| IBIS file stm32n657_vfbga198.ibs
[IBIS ver] 4.2
[File name] stm32n657_vfbga198.ibs
[File Rev] 1.1
[Date] 20-09-2024
[Source] Data Created at STMicroelectronics
[Notes]  File originated from ELDO simulations.
[Disclaimer]  This information is for modeling purpose only and is
   not guaranteed. The information is subject to change without
   notice.
[Copyright] Copyright 2024 STMicroelectronics Inc.
|   Component stm32n657_vfbga198
[Component] stm32n657_vfbga198
[Manufacturer] STMicroelectronics
[Package]
| variable   typ   min   max
R_pkg  0  NA  NA
L_pkg  0  NA  NA
C_pkg  0  NA  NA
[Pin]   signal_name   model_name
A1  PDR_ON  nc
A2  OTG2_HSDP  USB2_HS_IBIS
A3  NC  nc
A4  OTG1_HSDP  USB2_HS_IBIS
A5  PH0-OSC_IN  isudq_tt
A6  PC10  io8_tt_i3c
A7  PC7  io8_tt
A8  PE11  io8_tt
A9  PE15  io8_tt_i3c
A10  PD6  io8_tt
A11  PD12  io8_tt
A12  PD3  io8_tt_i3c
A13  PE10  io8_tt
A14  PB3  io8_tt
A15  VSS  gnd
B1  PC15-OSC32_OUT  io8_tt_sw
B2  OTG2_HSDM  USB2_HS_IBIS
B3  VDD33USB  power
B4  OTG1_HSDM  USB2_HS_IBIS
B5  PH1-OSC_OUT  isudq_tt
B6  PC9  io8_tt_i3c
B7  PC6  io8_tt
B8  PE14  io8_tt_i3c
B9  PE13  io8_tt_i3c
B10  PD7  io8_tt
B11  PD1  io8_tt
B12  PD4  io8_tt_i3c
B13  PD8  io8_tt
B14  PD11  io8_tt_i3c
B15  PE2  io8_tt
C1  PC14-OSC32_IN  io8_tt_sw
C2  NC  nc
C3  VDDA18USB  power
C4  OTG1_ID  nc
C5  OTG1_TXRTUNE  nc
C6  PC8  io8_tt_i3c
C7  PC1  io8_tt_i3c
C8  PE5  io8_tt_i3c
C9  PE12  io8_tt
C10  PD10  io8_tt
C11  PD0  io8_tt
C12  PE8  io8_tt
C13  PD5  io8_tt
C14  PE0  io8_tt
C15  PE3  io8_tt
D1  VBAT  power
D2  OTG2_ID  nc
D3  OTG2_TXRTUNE  nc
D4  UCPD1_CC1  nc
D5  UCPD1_CC2  nc
D6  PC11  io8_tt_i3c
D7  PH9  io8_tt_i3c
D8  PE6  io8_tt_i3c
D9  PD2  io8_tt
D10  PE7  io8_tt
D11  PD15  io8_tt_i3c
D12  PE9  io8_tt
D13  PE1  io8_tt
D14  PB6  io8_tt
D15  PB0  io8_tt
E1  V08CAP  nc
E2  VFBSMPS  nc
E3  BOOT0  isudq_tt
E4  NRST  ioreset_tt_v18_1v8
E5  VDDA18AON  nc
E6  PC12  io8_tt
E7  PH2  io8_tt
E8  VSS  gnd
E9  VDDIO4  power
E10  VDDIO4  power
E11  PD14  io8_tt_i3c
E12  PB7  io8_tt
E13  PD9  io8_tt
E14  PP2  io8_tt
E15  PP4  io8_tt
F1  VDDA18PMU  nc
F2  VSSAPMU  nc
F3  PWR_ON  io8_tt
F4  PC13  io8_tt_tamp
F5  VSSAON  nc
F11  PD13  io8_tt
F12  PO1  io8_tt
F13  PP3  io8_tt
F14  PO5  io8_tt
F15  PO4  io8_tt
G1  VSSSMPS  nc
G2  VSSSMPS  nc
G3  VSSSMPS  nc
G4  VSSSMPS  nc
G11  VSS  gnd
G12  PO0  io8_tt
G13  PP6  io8_tt
G14  PP0  io8_tt
G15  PP5  io8_tt
H1  VLXSMPS  nc
H2  VLXSMPS  nc
H3  VLXSMPS  nc
H4  VLXSMPS  nc
H11  VDD  power
H12  VDD  power
H13  PP1  io8_tt
H14  PP7  io8_tt
H15  PO2  io8_tt
J1  VDDSMPS  nc
J2  VDDSMPS  nc
J3  VDDSMPS  nc
J4  VDDSMPS  nc
J5  VDDA18PLL  nc
J11  VDDIO2  power
J12  VDDIO2  power
J13  VDD  power
J14  PN4  io8_tt
J15  PN8  io8_tt
K1  PF4  io8_tt
K2  PF6  io8_tt
K3  PF10  io8_tt
K4  PG6  io8_tt
K5  PG5  io8_tt
K11  VDDIO3  power
K12  PN1  io8_tt
K13  PN5  io8_tt
K14  PN7  io8_tt
K15  PN6  io8_tt
L1  PF5  io8_tt
L2  PF3  io8_tt
L3  PF2  io8_tt
L4  PF14  io8_tt
L5  VSS  gnd
L6  VDDCORE  nc
L7  VDDCORE  nc
L8  VDDCORE  nc
L9  VDDCORE  nc
L10  VSS  gnd
L11  VDDIO3  power
L12  PN12  io8_tt
L13  PN9  io8_tt
L14  PN2  io8_tt
L15  PN10  io8_tt
M1  PF15  io8_tt
M2  PF7  io8_tt
M3  PF8  io8_tt
M4  PF9  io8_tt
M5  VSSA  nc
M6  VDDA18ADC  nc
M7  PG15  io8_tt
M8  PG14  io8_tt
M9  PA9  io8_tt_i3c
M10  PA6  io8_tt_i3c
M11  PA1  io8_tt
M12  PB11  io8_tt_i3c
M13  PN0  io8_tt
M14  PN11  io8_tt
M15  PN3  io8_tt
N1  PF11  io8_tt
N2  PF1  io8_tt
N3  PF12  io8_tt
N4  PF0  io8_tt
N5  CSI_REXT  nc
N6  VDDCSI  nc
N7  PA12  io8_tt
N8  PA11  io8_tt
N9  PA8  io8_tt_i3c
N10  PG13  io8_tt
N11  PA0  io8_tt
N12  PB10  io8_tt_i3c
N13  PB4  io8_tt
N14  PG8  io8_tt
N15  PA3  io8_tt
P1  PF13  io8_tt
P2  PG4  io8_tt
P3  VREFM  nc
P4  CSI_D1N  DPHY_IBIS_L1
P5  CSI_CKN  DPHY_IBIS_L1
P6  CSI_D0N  DPHY_IBIS_L1
P7  VDDA18CSI  power
P8  PA10  io8_tt
P9  PA2  io8_tt
P10  PG12  io8_tt
P11  PG10  io8_tt
P12  PG2  io8_tt
P13  PA7  io8_tt
P14  PG11  io8_tt
P15  PG0  io8_tt
R1  VSS  gnd
R2  PG3  io8_tt
R3  VREFP  nc
R4  CSI_D1P  DPHY_IBIS_L1
R5  CSI_CKP  DPHY_IBIS_L1
R6  CSI_D0P  DPHY_IBIS_L1
R7  PA14  io8_tt
R8  PA13  io8_tt
R9  PA5  io8_tt_i3c
R10  PG1  io8_tt
R11  PB12  io8_tt_i3c
R12  PB5  io8_tt_i3c
R13  PA15  io8_tt
R14  PG9  io8_tt
R15  VSS  gnd
[Package Model]   486-fcvfbga-10x10-198-240308
[Pin Mapping]   pulldown_ref   pullup_ref   | Comment
A1  nc  nc
A2  gnd  VDD33USB
A3  nc  nc
A4  gnd  VDD33USB
A5  gnd  VDD
A6  gnd  VDDIO4
A7  gnd  VDDIO4
A8  gnd  VDD
A9  gnd  VDD
A10  gnd  VDD
A11  gnd  VDD
A12  gnd  VDD
A13  gnd  VDD
A14  gnd  VDD
A15  gnd  nc
B1  gnd  VSW
B2  gnd  VDD33USB
B3  nc  VDD33USB
B4  gnd  VDD33USB
B5  gnd  VDD
B6  gnd  VDDIO4
B7  gnd  VDDIO4
B8  gnd  VDD
B9  gnd  VDD
B10  gnd  VDD
B11  gnd  VDD
B12  gnd  VDD
B13  gnd  VDD
B14  gnd  VDD
B15  gnd  VDD
C1  gnd  VSW
C2  nc  nc
C3  nc  VDDA18USB
C4  nc  nc
C5  nc  nc
C6  gnd  VDDIO4
C7  gnd  VDDIO4
C8  gnd  VDD
C9  gnd  VDD
C10  gnd  VDD
C11  gnd  VDD
C12  gnd  VDD
C13  gnd  VDD
C14  gnd  VDD
C15  gnd  VDD
D1  nc  VSW
D2  nc  nc
D3  nc  nc
D4  nc  nc
D5  nc  nc
D6  gnd  VDDIO4
D7  gnd  VDDIO4
D8  gnd  VDD
D9  gnd  VDD
D10  gnd  VDD
D11  gnd  VDD
D12  gnd  VDD
D13  gnd  VDD
D14  gnd  VDD
D15  gnd  VDD
E1  nc  nc
E2  nc  nc
E3  gnd  VDD
E4  gnd  VDD
E5  nc  nc
E6  gnd  VDDIO4
E7  gnd  VDDIO4
E8  gnd  nc
E9  nc  VDDIO4
E10  nc  VDDIO4
E11  gnd  VDD
E12  gnd  VDD
E13  gnd  VDD
E14  gnd  VDDIO2
E15  gnd  VDDIO2
F1  nc  nc
F2  nc  nc
F3  gnd  VDD
F4  gnd  VSW
F5  nc  nc
F11  gnd  VDD
F12  gnd  VDDIO2
F13  gnd  VDDIO2
F14  gnd  VDDIO2
F15  gnd  VDDIO2
G1  nc  nc
G2  nc  nc
G3  nc  nc
G4  nc  nc
G11  gnd  nc
G12  gnd  VDDIO2
G13  gnd  VDDIO2
G14  gnd  VDDIO2
G15  gnd  VDDIO2
H1  nc  nc
H2  nc  nc
H3  nc  nc
H4  nc  nc
H11  nc  VDD
H12  nc  VDD
H13  gnd  VDDIO2
H14  gnd  VDDIO2
H15  gnd  VDDIO2
J1  nc  nc
J2  nc  nc
J3  nc  nc
J4  nc  nc
J5  nc  nc
J11  nc  VDDIO2
J12  nc  VDDIO2
J13  nc  VDD
J14  gnd  VDDIO3
J15  gnd  VDDIO3
K1  gnd  VDD
K2  gnd  VDD
K3  gnd  VDD
K4  gnd  VDD
K5  gnd  VDD
K11  nc  VDDIO3
K12  gnd  VDDIO3
K13  gnd  VDDIO3
K14  gnd  VDDIO3
K15  gnd  VDDIO3
L1  gnd  VDD
L2  gnd  VDD
L3  gnd  VDD
L4  gnd  VDD
L5  gnd  nc
L6  nc  nc
L7  nc  nc
L8  nc  nc
L9  nc  nc
L10  gnd  nc
L11  nc  VDDIO3
L12  gnd  VDDIO3
L13  gnd  VDDIO3
L14  gnd  VDDIO3
L15  gnd  VDDIO3
M1  gnd  VDD
M2  gnd  VDD
M3  gnd  VDD
M4  gnd  VDD
M5  nc  nc
M6  nc  nc
M7  gnd  VDD
M8  gnd  VDD
M9  gnd  VDD
M10  gnd  VDD
M11  gnd  VDD
M12  gnd  VDD
M13  gnd  VDDIO3
M14  gnd  VDDIO3
M15  gnd  VDDIO3
N1  gnd  VDD
N2  gnd  VDD
N3  gnd  VDD
N4  gnd  VDD
N5  nc  nc
N6  nc  nc
N7  gnd  VDD
N8  gnd  VDD
N9  gnd  VDD
N10  gnd  VDD
N11  gnd  VDD
N12  gnd  VDD
N13  gnd  VDD
N14  gnd  VDD
N15  gnd  VDD
P1  gnd  VDD
P2  gnd  VDD
P3  nc  nc
P4  gnd  VDDA18CSI
P5  gnd  VDDA18CSI
P6  gnd  VDDA18CSI
P7  nc  VDDA18CSI
P8  gnd  VDD
P9  gnd  VDD
P10  gnd  VDD
P11  gnd  VDD
P12  gnd  VDD
P13  gnd  VDD
P14  gnd  VDD
P15  gnd  VDD
R1  gnd  nc
R2  gnd  VDD
R3  nc  nc
R4  gnd  VDDA18CSI
R5  gnd  VDDA18CSI
R6  gnd  VDDA18CSI
R7  gnd  VDD
R8  gnd  VDD
R9  gnd  VDD
R10  gnd  VDD
R11  gnd  VDD
R12  gnd  VDD
R13  gnd  VDD
R14  gnd  VDD
R15  gnd  nc
[Diff Pin]  inv_pin  vdiff  tdelay_typ  tdelay_min  tdelay_max
R5  P5  NA  NA  NA  NA
R6  P6  NA  NA  NA  NA
R4  P4  NA  NA  NA  NA
A4  B4  NA  NA  NA  NA
A2  B2  NA  NA  NA  NA
[Model Selector] DPHY_IBIS_L1
DPHY_RX_2P5G_L1   DPHY HSRX model at 2.5Gbps for lane 1
DPHY_RX_1P5G_L1   DPHY HSRX model at 1.5Gbps for lane 1
[Model Selector] io8_tt
io8_tt_ls_3v3 "GPIO - 3V tolerant - low speed - 3.3V range"
io8_tt_ms_3v3 "GPIO - 3V tolerant - med speed - 3.3V range"
io8_tt_fs_3v3 "GPIO - 3V tolerant - fast speed - 3.3V range"
io8_tt_hs_3v3 "GPIO - 3V tolerant - high speed - 3.3V range"
io8_tt_hslv_ls_1v8 "GPIO low voltage optimization - 3V tolerant - low speed - 1.8V range"
io8_tt_hslv_ms_1v8 "GPIO low voltage optimization - 3V tolerant - med speed - 1.8V range"
io8_tt_hslv_fs_1v8 "GPIO low voltage optimization - 3V tolerant - fast speed - 1.8V range"
io8_tt_hslv_hs_1v8 "GPIO low voltage optimization - 3V tolerant - high speed - 1.8V range"
[Model Selector] io8_tt_i3c
io8_tt_ls_3v3 "GPIO - 3V tolerant - low speed - 3.3V range"
io8_tt_ms_3v3 "GPIO - 3V tolerant - med speed - 3.3V range"
io8_tt_fs_3v3 "GPIO - 3V tolerant - fast speed - 3.3V range"
io8_tt_hs_3v3 "GPIO - 3V tolerant - high speed - 3.3V range"
io8_tt_hslv_ls_1v8 "GPIO low voltage optimization - 3V tolerant - low speed - 1.8V range"
io8_tt_hslv_ms_1v8 "GPIO low voltage optimization - 3V tolerant - med speed - 1.8V range"
io8_tt_hslv_fs_1v8 "GPIO low voltage optimization - 3V tolerant - fast speed - 1.8V range"
io8_tt_hslv_hs_1v8 "GPIO low voltage optimization - 3V tolerant - high speed - 1.8V range"
io8_tt_i3c_ls_3v3 "GPIO with I3C open-drain - 3V tolerant - low speed - 3.3V range"
io8_tt_i3c_ms_3v3 "GPIO with I3C open-drain - 3V tolerant - med speed - 3.3V range"
io8_tt_i3c_fs_3v3 "GPIO with I3C open-drain - 3V tolerant - fast speed - 3.3V range"
io8_tt_i3c_hs_3v3 "GPIO with I3C open-drain - 3V tolerant - high speed - 3.3V range"
io8_tt_hslv_i3c_ls_1v8 "GPIO low voltage optimization with I3C open-drain - 3V tolerant - low speed - 1.8V range"
io8_tt_hslv_i3c_ms_1v8 "GPIO low voltage optimization with I3C open-drain - 3V tolerant - med speed - 1.8V range"
io8_tt_hslv_i3c_fs_1v8 "GPIO low voltage optimization with I3C open-drain - 3V tolerant - fast speed - 1.8V range"
io8_tt_hslv_i3c_hs_1v8 "GPIO low voltage optimization with I3C open-drain - 3V tolerant - high speed - 1.8V range"
io8_tt_i3c_fmp_3v3 "GPIO with I3C fm+ open-drain - 3V tolerant - 3.3V range"
[Model Selector] io8_tt_sw
io8_tt_sw_3v3 "Input Buffer - 3V tolerant - 3.3V range"
io8_tt_sw_1v8 "Input Buffer - 3V tolerant - 1.8V range"
[Model Selector] io8_tt_tamp
io8_tt_ls_3v3 "GPIO - 3V tolerant - low speed - 3.3V range"
io8_tt_ms_3v3 "GPIO - 3V tolerant - med speed - 3.3V range"
io8_tt_fs_3v3 "GPIO - 3V tolerant - fast speed - 3.3V range"
io8_tt_hs_3v3 "GPIO - 3V tolerant - high speed - 3.3V range"
io8_tt_hslv_ls_1v8 "GPIO low voltage optimization - 3V tolerant - low speed - 1.8V range"
io8_tt_hslv_ms_1v8 "GPIO low voltage optimization - 3V tolerant - med speed - 1.8V range"
io8_tt_hslv_fs_1v8 "GPIO low voltage optimization - 3V tolerant - fast speed - 1.8V range"
io8_tt_hslv_hs_1v8 "GPIO low voltage optimization - 3V tolerant - high speed - 1.8V range"
io8_tt_tamp_3v3 "IO tamper - 3V tolerant - 3.3V range"
io8_tt_tamp_1v8 "IO tamper - 3V tolerant - 1.8V range"
|[Model Selector] ioreset_tt_v18
|ioreset_tt_v18_1v8 "Reset PAD - 3V tolerant - 1.8V range"
[Model Selector] isudq_tt
isudq_tt_3v3 "Input Buffer - 3V tolerant - 3.3V range"
isudq_tt_1v8 "Input Buffer - 3V tolerant - 1.8V range"
[Model Selector] USB2_HS_IBIS
USB2_HSRX   USB2 HSRX model
USB2_HSTX_00_0_01_0011_11   TuningBits_AMP_PULSE_RISE_REF_XV=00_0_01_0011_11
USB2_HSTX_00_0_10_0101_11   TuningBits_AMP_PULSE_RISE_REF_XV=00_0_10_0101_11
USB2_HSTX_00_0_11_0111_11   TuningBits_AMP_PULSE_RISE_REF_XV=00_0_11_0111_11
USB2_HSTX_00_1_01_0011_11   TuningBits_AMP_PULSE_RISE_REF_XV=00_1_01_0011_11
USB2_HSTX_00_1_10_0101_11   TuningBits_AMP_PULSE_RISE_REF_XV=00_1_10_0101_11
USB2_HSTX_00_1_11_0111_11   TuningBits_AMP_PULSE_RISE_REF_XV=00_1_11_0111_11
USB2_HSTX_01_0_01_0011_11   TuningBits_AMP_PULSE_RISE_REF_XV=01_0_01_0011_11
USB2_HSTX_01_0_10_0101_11   TuningBits_AMP_PULSE_RISE_REF_XV=01_0_10_0101_11
USB2_HSTX_01_0_11_0111_11   TuningBits_AMP_PULSE_RISE_REF_XV=01_0_11_0111_11
USB2_HSTX_01_1_01_0011_11   TuningBits_AMP_PULSE_RISE_REF_XV=01_1_01_0011_11
USB2_HSTX_01_1_10_0101_11   TuningBits_AMP_PULSE_RISE_REF_XV=01_1_10_0101_11
USB2_HSTX_01_1_11_0111_11   TuningBits_AMP_PULSE_RISE_REF_XV=01_1_11_0111_11
USB2_HSTX_10_0_01_0011_11   TuningBits_AMP_PULSE_RISE_REF_XV=10_0_01_0011_11
USB2_HSTX_10_0_10_0101_11   TuningBits_AMP_PULSE_RISE_REF_XV=10_0_10_0101_11
USB2_HSTX_10_0_11_0111_11   TuningBits_AMP_PULSE_RISE_REF_XV=10_0_11_0111_11
USB2_HSTX_10_1_01_0011_11   TuningBits_AMP_PULSE_RISE_REF_XV=10_1_01_0011_11
USB2_HSTX_10_1_10_0101_11   TuningBits_AMP_PULSE_RISE_REF_XV=10_1_10_0101_11
USB2_HSTX_10_1_11_0111_11   TuningBits_AMP_PULSE_RISE_REF_XV=10_1_11_0111_11
[Define Package Model]  486-fcvfbga-10x10-198-240308
[Manufacturer]  unknown
[OEM]  unknown
[Description]  unknown
[Number Of Pins]  175
[Pin Numbers]
| Pin Name Terminal   Net Name   Starting Node   Ending Node
E3 | BOOT0
P5 | CSI_CKN
R5 | CSI_CKP
P6 | CSI_D0N
R6 | CSI_D0P
P4 | CSI_D1N
R4 | CSI_D1P
N5 | CSI_REXT
E4 | NRST
B4 | OTG1_HSDM
A4 | OTG1_HSDP
C4 | OTG1_ID
C5 | OTG1_TXRTUNE
A3 | NC
B2 | OTG2_HSDM
A2 | OTG2_HSDP
D2 | OTG2_ID
D3 | OTG2_TXRTUNE
C2 | NC
N11 | PA0
M11 | PA1
P9 | PA2
N15 | PA3
R9 | PA5
M10 | PA6
P13 | PA7
N9 | PA8
M9 | PA9
P8 | PA10
N8 | PA11
N7 | PA12
R8 | PA13
R7 | PA14
R13 | PA15
D15 | PB0
A14 | PB3
N13 | PB4
R12 | PB5
D14 | PB6
E12 | PB7
N12 | PB10
M12 | PB11
R11 | PB12
C7 | PC1
B7 | PC6
A7 | PC7
C6 | PC8
B6 | PC9
A6 | PC10
D6 | PC11
E6 | PC12
F4 | PC13
C1 | PC14-OSC32_IN
B1 | PC15-OSC32_OUT
C11 | PD0
B11 | PD1
D9 | PD2
A12 | PD3
B12 | PD4
C13 | PD5
A10 | PD6
B10 | PD7
B13 | PD8
E13 | PD9
C10 | PD10
B14 | PD11
A11 | PD12
F11 | PD13
E11 | PD14
D11 | PD15
A1 | PDR_ON
C14 | PE0
D13 | PE1
B15 | PE2
C15 | PE3
C8 | PE5
D8 | PE6
D10 | PE7
C12 | PE8
D12 | PE9
A13 | PE10
A8 | PE11
C9 | PE12
B9 | PE13
B8 | PE14
A9 | PE15
N4 | PF0
N2 | PF1
L3 | PF2
L2 | PF3
K1 | PF4
L1 | PF5
K2 | PF6
M2 | PF7
M3 | PF8
M4 | PF9
K3 | PF10
N1 | PF11
N3 | PF12
P1 | PF13
L4 | PF14
M1 | PF15
P15 | PG0
R10 | PG1
P12 | PG2
R2 | PG3
P2 | PG4
K5 | PG5
K4 | PG6
N14 | PG8
R14 | PG9
P11 | PG10
P14 | PG11
P10 | PG12
N10 | PG13
M8 | PG14
M7 | PG15
A5 | PH0-OSC_IN
B5 | PH1-OSC_OUT
E7 | PH2
D7 | PH9
M13 | PN0
K12 | PN1
L14 | PN2
M15 | PN3
J14 | PN4
K13 | PN5
K15 | PN6
K14 | PN7
J15 | PN8
L13 | PN9
L15 | PN10
M14 | PN11
L12 | PN12
G12 | PO0
F12 | PO1
H15 | PO2
F15 | PO4
F14 | PO5
G14 | PP0
H13 | PP1
E14 | PP2
F13 | PP3
E15 | PP4
G15 | PP5
G13 | PP6
H14 | PP7
F3 | PWR_ON
D4 | UCPD1_CC1
D5 | UCPD1_CC2
E1 | V08CAP
D1 | VBAT
B3 | VDD33USB
H11 | VDD
M6 | VDDA18ADC
E5 | VDDA18AON
P7 | VDDA18CSI
J5 | VDDA18PLL
F1 | VDDA18PMU
C3 | VDDA18USB
L6 | VDDCORE
N6 | VDDCSI
J11 | VDDIO2
K11 | VDDIO3
E9 | VDDIO4
J1 | VDDSMPS
E2 | VFBSMPS
H1 | VLXSMPS
P3 | VREFM
R3 | VREFP
A15 | VSS
M5 | VSSA
F5 | VSSAON
F2 | VSSAPMU
G1 | VSSSMPS
|[Merged Pins]  H11
|H12  |  VDD
|J13  |  VDD
|[Merged Pins]  L6
|L7  |  VDDCORE
|L8  |  VDDCORE
|L9  |  VDDCORE
|[Merged Pins]  J11
|J12  |  VDDIO2
|[Merged Pins]  K11
|L11  |  VDDIO3
|[Merged Pins]  E9
|E10  |  VDDIO4
|[Merged Pins]  J1
|J2  |  VDDSMPS
|J3  |  VDDSMPS
|J4  |  VDDSMPS
|[Merged Pins]  H1
|H2  |  VLXSMPS
|H3  |  VLXSMPS
|H4  |  VLXSMPS
|[Merged Pins]  A15
|E8  |  VSS
|G11  |  VSS
|L5  |  VSS
|L10  |  VSS
|R1  |  VSS
|R15  |  VSS
|[Merged Pins]  G1
|G2  |  VSSSMPS
|G3  |  VSSSMPS
|G4  |  VSSSMPS
[Model Data]
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[End Model Data]
[End Package Model]
|End [Component]
| Models and submodels in the file (45): DPHY_RX_1P5G_L1 (Input), DPHY_RX_2P5G_L1 (Input), io8_tt_fs_3v3 (I/O), io8_tt_hs_3v3 (I/O), io8_tt_hslv_fs_1v8 (I/O), io8_tt_hslv_hs_1v8 (I/O), io8_tt_hslv_i3c_fs_1v8 (I/O_open_drain), io8_tt_hslv_i3c_hs_1v8 (I/O_open_drain), io8_tt_hslv_i3c_ls_1v8 (I/O_open_drain), io8_tt_hslv_i3c_ms_1v8 (I/O_open_drain), io8_tt_hslv_ls_1v8 (I/O), io8_tt_hslv_ms_1v8 (I/O), io8_tt_i3c_fmp_3v3 (I/O_open_drain), io8_tt_i3c_fs_3v3 (I/O_open_drain), io8_tt_i3c_hs_3v3 (I/O_open_drain), io8_tt_i3c_ls_3v3 (I/O_open_drain), io8_tt_i3c_ms_3v3 (I/O_open_drain), io8_tt_ls_3v3 (I/O), io8_tt_ms_3v3 (I/O), io8_tt_sw_1v8 (I/O), io8_tt_sw_3v3 (I/O), io8_tt_tamp_1v8 (I/O), io8_tt_tamp_3v3 (I/O), ioreset_tt_v18_1v8 (I/O_open_drain), isudq_tt_1v8 (Input), isudq_tt_3v3 (Input), USB2_HSRX (Input), USB2_HSTX_00_0_01_0011_11 (Output), USB2_HSTX_00_0_10_0101_11 (Output), USB2_HSTX_00_0_11_0111_11 (Output), USB2_HSTX_00_1_01_0011_11 (Output), USB2_HSTX_00_1_10_0101_11 (Output), USB2_HSTX_00_1_11_0111_11 (Output), USB2_HSTX_01_0_01_0011_11 (Output), USB2_HSTX_01_0_10_0101_11 (Output), USB2_HSTX_01_0_11_0111_11 (Output), USB2_HSTX_01_1_01_0011_11 (Output), USB2_HSTX_01_1_10_0101_11 (Output), USB2_HSTX_01_1_11_0111_11 (Output), USB2_HSTX_10_0_01_0011_11 (Output), USB2_HSTX_10_0_10_0101_11 (Output), USB2_HSTX_10_0_11_0111_11 (Output), USB2_HSTX_10_1_01_0011_11 (Output), USB2_HSTX_10_1_10_0101_11 (Output), USB2_HSTX_10_1_11_0111_11 (Output)
